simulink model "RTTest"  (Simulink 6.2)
settings: Solver=FixedStepDiscrete  StartTime=0.0  StopTime=inf  RelTol=1e-3
PreLoadFcn:
  | initialize
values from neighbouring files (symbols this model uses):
  nAcc = 1    [initialize.m]
  nAdcU = 6    [initialize.m]    (also in Copy of initialize.m)
  node = completenodestruct(node)    [initialize.m]    (also in Copy of initialize.m)
libraries: xpclib x5

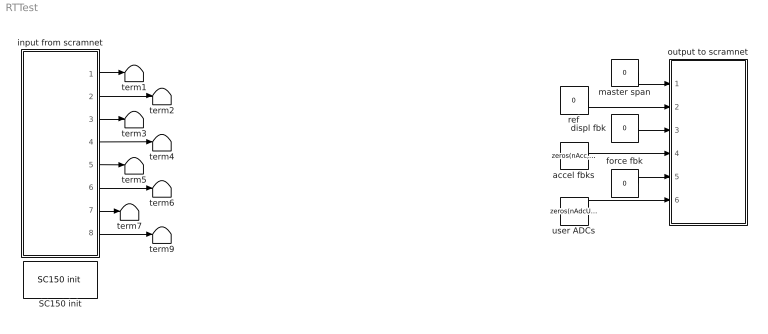
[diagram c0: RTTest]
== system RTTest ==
  SC150 init : xpclib/Shared Memory/Systran/SC150 init   node=node  pci=-1
  accel fbks : Constant  Value=zeros(nAcc,1)
  displ fbk : Constant  Value=0
  force fbk : Constant  Value=0
  input from scramnet : Subsystem
  master span : Constant  Value=0
  output to scramnet : Subsystem
  ref : Constant  Value=0
  term{1..7,9} (8 alike) : Terminator
  user ADCs : Constant  Value=zeros(nAdcU, 1)
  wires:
  input from scramnet/1(master span) -> term1/1
  input from scramnet/2(ref) -> term2/1
  input from scramnet/3(displ fbk) -> term3/1
  input from scramnet/4(veloc fbk) -> term4/1
  input from scramnet/5(accel fbk) -> term5/1
  input from scramnet/6(force fbk) -> term6/1
  input from scramnet/8(user adcs) -> term9/1
  input from scramnet/7(valve cmd) -> term7/1
  user ADCs/1 -> output to scramnet/6(user adcs)
  master span/1 -> output to scramnet/1(master span)
  ref/1 -> output to scramnet/2(ref)
  displ fbk/1 -> output to scramnet/3(displ fbk)
  accel fbks/1 -> output to scramnet/4(accel fbk)
  force fbk/1 -> output to scramnet/5(force fbk)

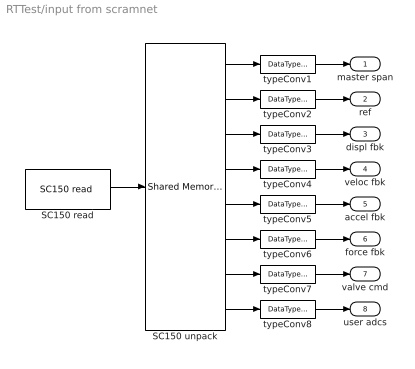
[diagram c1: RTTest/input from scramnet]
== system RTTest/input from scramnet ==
  SC150 read : xpclib/Shared Memory/Systran/SC150 read   partition=node.Partitions(7:14)  ts=samplePeriod  pci=-1
  SC150 unpack : xpclib/Shared Memory/Shared Memory Unpack   partition=node.Partitions(7:14)
  typeConv{1..8} (8 alike) : DataTypeConversion  OutDataTypeMode=double
  master span : Outport
  ref : Outport  Port=2
  displ fbk : Outport  Port=3
  veloc fbk : Outport  Port=4
  accel fbk : Outport  Port=5
  force fbk : Outport  Port=6
  valve cmd : Outport  Port=7
  user adcs : Outport  Port=8
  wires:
  SC150 read/1 -> SC150 unpack/1
  typeConv1/1 -> master span/1
  typeConv2/1 -> ref/1
  typeConv3/1 -> displ fbk/1
  typeConv4/1 -> veloc fbk/1
  typeConv5/1 -> accel fbk/1
  typeConv6/1 -> force fbk/1
  typeConv7/1 -> valve cmd/1
  typeConv8/1 -> user adcs/1
  SC150 unpack/1 -> typeConv1/1
  SC150 unpack/2 -> typeConv2/1
  SC150 unpack/3 -> typeConv3/1
  SC150 unpack/4 -> typeConv4/1
  SC150 unpack/5 -> typeConv5/1
  SC150 unpack/6 -> typeConv6/1
  SC150 unpack/7 -> typeConv7/1
  SC150 unpack/8 -> typeConv8/1

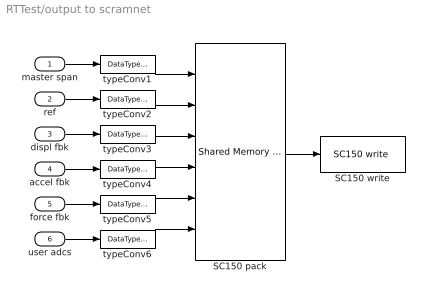
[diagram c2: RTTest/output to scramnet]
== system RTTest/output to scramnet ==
  master span : Inport  Port=1  LatchInput=off
  ref : Inport  Port=2  LatchInput=off
  displ fbk : Inport  Port=3  LatchInput=off
  accel fbk : Inport  Port=4  LatchInput=off
  force fbk : Inport  Port=5  LatchInput=off
  user adcs : Inport  Port=6  LatchInput=off
  SC150 pack : xpclib/Shared Memory/Shared Memory Pack   partition=node.Partitions(1:6)
  SC150 write : xpclib/Shared Memory/Systran/SC150 write   partition=node.Partitions(1:6)  ts=samplePeriod  pci=-1
  typeConv{1..6} (6 alike) : DataTypeConversion  OutDataTypeMode=single
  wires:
  master span/1 -> typeConv1/1
  ref/1 -> typeConv2/1
  displ fbk/1 -> typeConv3/1
  accel fbk/1 -> typeConv4/1
  SC150 pack/1 -> SC150 write/1
  typeConv1/1 -> SC150 pack/1
  typeConv2/1 -> SC150 pack/2
  typeConv3/1 -> SC150 pack/3
  typeConv4/1 -> SC150 pack/4
  force fbk/1 -> typeConv5/1
  user adcs/1 -> typeConv6/1
  typeConv5/1 -> SC150 pack/5
  typeConv6/1 -> SC150 pack/6
